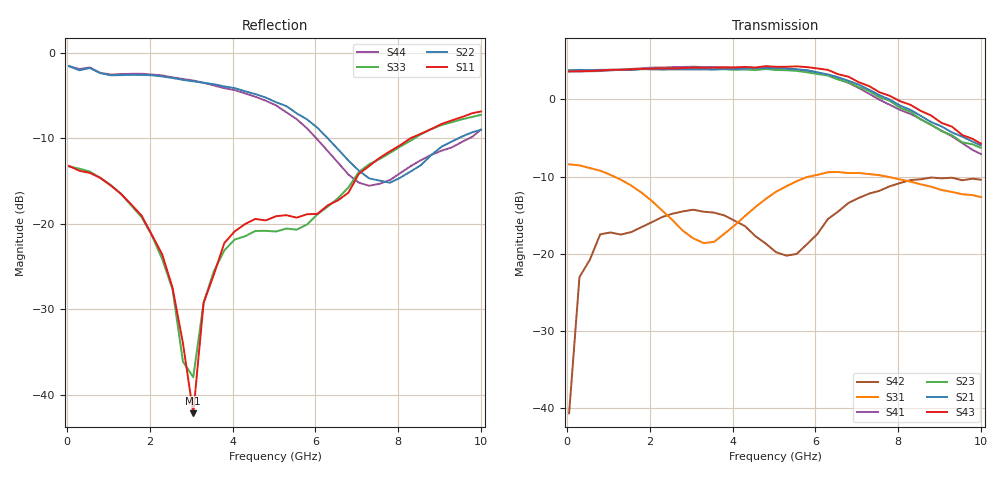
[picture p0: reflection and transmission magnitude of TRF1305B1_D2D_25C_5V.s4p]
! Created Tue Jun 24 22:54:35 2025
# hz S ma R 50
! 4 Port Network Data from SP1.SP block
! PORT[1] = INP
! PORT[2] = OUTM
! PORT[3] = INM
! PORT[4] = OUTP
! freq  magS11  angS11  magS12  angS12  magS13  angS13  magS14  angS14
!  magS21  angS21  magS22  angS22  magS23  angS23  magS24  angS24
!  magS31  angS31  magS32  angS32  magS33  angS33  magS34  angS34
!  magS41  angS41  magS42  angS42  magS43  angS43  magS44  angS44
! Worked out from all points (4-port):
!   41 points, 50 MHz to 10 GHz, reference 50 ohm
!   strongest paths, dB at 50 MHz, 2.55 GHz, 5.05 GHz, 7.55 GHz, 10 GHz:
!     S43: 3.6, 4.0, 4.2, 0.9, -5.7
!     S21: 3.8, 3.9, 4.1, 0.6, -6.0
!     S23: 3.8, 4.0, 3.8, 0.3, -6.3
!     S41: 3.6, 4.2, 4.1, 0.0, -7.1
!     S31: -8.4, -15.7, -12.0, -9.8, -12.7
!     S42: -40.7, -14.8, -19.8, -11.8, -10.4
!   lowest |S11| = -42.2 dB at 3.05 GHz (marker M1), VSWR 1.02, Z = 50.2 + j0.753 ohm
!   |S11| at or under -10 dB: start of sweep to 8.295 GHz
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5e7  0.218 -1.9  0.0024 -6.6  0.3811 -2.3  0.0035 98.9
     1.545 178.2  0.8365 178.6  1.546 -2.2  0.01037 113.6
     0.3796 -2.3  0.0005635 151.7  0.2165 -1.4  0.003508 131.8
     1.518 -2.1  0.009213 95.1  1.52 177.5  0.837 178.8
3e8  0.204 -13.2  0.01545 47.5  0.3708 -12.8  0.008462 57.0
     1.555 168.7  0.7922 170.6  1.522 -12.0  0.06806 59.1
     0.3737 -12.7  0.01312 52.5  0.21 -13.3  0.01453 51.5
     1.522 -11.9  0.07056 58.4  1.525 168.0  0.8049 171.9
3.05e9  0.007761 75.1  0.05684 -26.2  0.1208 -153.3  0.03752 -46.8
        1.564 53.8  0.6825 115.2  1.581 -123.6  0.1921 -11.5
        0.1257 -155.3  0.03938 -55.5  0.01262 44.1  0.05914 -20.9
        1.631 -122.2  0.1927 -14.6  1.61 55.7  0.6899 119.8
4.55e9  0.1067 30.3  0.06398 -65.7  0.1951 92.8  0.04088 -108.4
        1.597 -10.4  0.5746 84.7  1.55 172.3  0.1301 -74.1
        0.2003 90.3  0.04215 -114.0  0.09072 32.4  0.06994 -64.3
        1.599 172.6  0.1299 -80.8  1.612 -7.9  0.5546 89.2
6.05e9  0.1142 14.3  0.07715 -105.3  0.3342 35.9  0.03312 178.8
        1.5 -82.7  0.3649 50.2  1.463 98.4  0.1157 133.4
        0.3244 33.0  0.02933 178.0  0.1136 26.8  0.08342 -105.4
        1.493 99.2  0.1341 133.0  1.589 -80.8  0.3116 58.5
7.3e9  0.2178 25.1  0.079 -146.6  0.3446 -1.0  0.01304 129.0
       1.155 -144.3  0.1843 66.1  1.134 36.2  0.2382 65.4
       0.3281 -1.9  0.01446 142.2  0.2229 29.0  0.08571 -145.3
       1.088 36.2  0.2451 66.7  1.22 -141.1  0.1668 72.9
1e10  0.4542 -45.4  0.06268 138.1  0.2359 -46.2  0.002923 138.8
      0.5039 113.9  0.3545 76.9  0.4856 -73.6  0.3045 -2.6
      0.2328 -43.8  0.008033 105.3  0.4343 -41.7  0.0682 139.5
      0.443 -70.6  0.3018 -1.1  0.5171 114.7  0.3561 76.6
